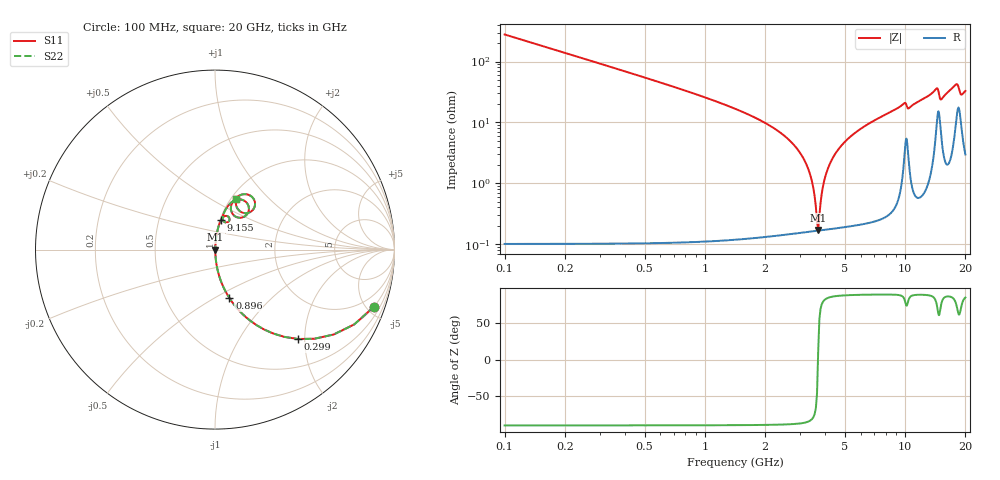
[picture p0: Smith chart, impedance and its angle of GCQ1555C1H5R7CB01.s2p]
!Murata Part Number: GCQ1555C1H5R7CB01
!These Parameters are Measured in Series Mode Connection
!Data Generated on Mar 13, 2026
!  o--ll--o
!Port1  Port2
!  o------o
!Operation Temp=25[degC], DC Bias Voltage=0[V]
!Freq. Start=100[MHz] Stop=20[GHz] 401[Steps]
# Hz S RI R 50
!Freq.(Hz) S11(Real) S11(Imag) S21(Real) S21(Imag) S12(Real) S12(Imag) S22(Real) S22(Imag)
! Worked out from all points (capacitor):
!   401 points, 100 MHz to 20 GHz, reference 50 ohm
!   read as one part in series: C = 5.7 pF near 199.5 MHz
!   lowest |Z| = 170 mohm at 3.682 GHz (marker M1)
!   series resonance near 3.673 GHz, so ESL is about 330 pH
!   S11 on the Smith chart (normalised r, x): 100 MHz: 1.00, -5.58; 299 MHz: 1.00, -1.86; 896 MHz: 1.00, -0.59; 9.155 GHz: 1.01, +0.34; 20 GHz: 1.06, +0.66
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1e8  0.8861 -0.3175  0.1139 0.3175  0.1139 0.3175  0.8861 -0.3175
2.99e8  0.4626 -0.498  0.5374 0.498  0.5374 0.498  0.4626 -0.498
5.4775e8  0.1995 -0.3986  0.8005 0.3986  0.8005 0.3986  0.1995 -0.3986
8.96e8  0.0799 -0.2693  0.9201 0.2693  0.9201 0.2693  0.0799 -0.2693
2.7865e9  0.00328 -0.0423  0.9967 0.0423  0.9967 0.0423  0.00328 -0.0423
3.1845e9  0.00204 -0.0217  0.998 0.0217  0.998 0.0217  0.00204 -0.0217
3.43325e9  0.00172 -0.0103  0.9983 0.0103  0.9983 0.0103  0.00172 -0.0103
3.5825e9  0.00166 -0.0038  0.9983 0.0038  0.9983 0.0038  0.00166 -0.0038
3.682e9  0.00166 0.000362  0.9983 -0.000362  0.9983 -0.000362  0.00166 0.000362
4.03025e9  0.00193 0.0141  0.9981 -0.0141  0.9981 -0.0141  0.00193 0.0141
4.478e9  0.00273 0.0303  0.9973 -0.0303  0.9973 -0.0303  0.00273 0.0303
5.3735e9  0.0055 0.0593  0.9945 -0.0593  0.9945 -0.0593  0.0055 0.0593
6.7665e9  0.0122 0.0991  0.9878 -0.0991  0.9878 -0.0991  0.0122 0.0991
9.1545e9  0.0329 0.1646  0.9671 -0.1646  0.9671 -0.1646  0.0329 0.1646
1.005e10  0.0787 0.1784  0.9213 -0.1784  0.9213 -0.1784  0.0787 0.1784
1.338325e10  0.0873 0.2595  0.9127 -0.2595  0.9127 -0.2595  0.0873 0.2595
1.437825e10  0.1704 0.2672  0.8296 -0.2672  0.8296 -0.2672  0.1704 0.2672
1.507475e10  0.1066 0.1895  0.8934 -0.1895  0.8934 -0.1895  0.1066 0.1895
1.67165e10  0.117 0.2888  0.883 -0.2888  0.883 -0.2888  0.117 0.2888
1.83085e10  0.2231 0.2534  0.7769 -0.2534  0.7769 -0.2534  0.2231 0.2534
1.895525e10  0.1469 0.2086  0.8531 -0.2086  0.8531 -0.2086  0.1469 0.2086
2e10  0.1184 0.2809  0.8816 -0.2809  0.8816 -0.2809  0.1184 0.2809
